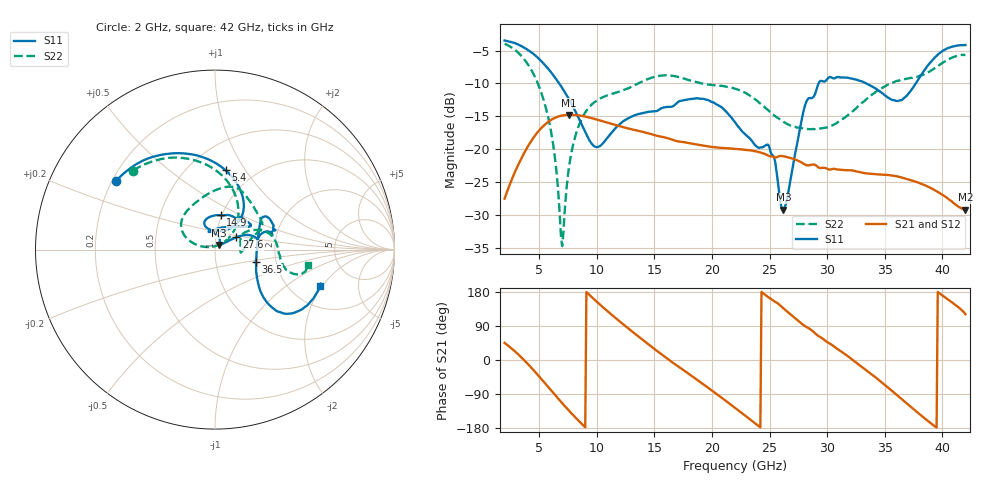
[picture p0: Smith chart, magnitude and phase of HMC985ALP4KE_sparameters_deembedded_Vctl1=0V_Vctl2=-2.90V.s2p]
!s2p File: Measurements: S11, S21, S12, S22
# GHz S dB R 50.0
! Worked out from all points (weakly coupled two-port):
!   401 points, 2 GHz to 42 GHz, reference 50 ohm
!   highest |S21| = -14.78 dB at 7.6 GHz (marker M1); lowest = -29.2 dB at 42 GHz (marker M2)
!   lowest |S11| = -29.2 dB at 26.2 GHz (marker M3), VSWR 1.07, Z = 52.3 + j2.72 ohm
!   |S11| at or under -10 dB: 6.736 GHz to 29.26 GHz (22.52 GHz wide, 125 % of centre); 33.39 GHz to 37.7 GHz (4.308 GHz wide, 12.1 % of centre)
!   |S22| runs from -34.8 to -4.0 dB; largest |S21 - S12| = 0.00076
!   S11 on the Smith chart (normalised r, x): 2 GHz: 0.22, +0.30; 5.4 GHz: 0.74, +0.82; 14.9 GHz: 0.99, +0.39; 27.6 GHz: 1.26, +0.18; 36.5 GHz: 1.57, -0.22; 42 GHz: 2.92, -1.90
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2  -3.47 145.0  -27.53 45.1  -27.52 45.1  -3.97 136.0
3.5  -4.37 118.8  -21.26 5.5  -21.27 5.4  -5.92 102.0
5.4  -7.01 82.5  -16.42 -57.7  -16.44 -57.7  -12.61 56.2
6.3  -8.92 66.5  -15.29 -89.6  -15.27 -89.6  -20.36 40.1
6.9  -10.44 57.8  -14.92 -110.6  -14.94 -110.6  -33.41 74.2
7.1  -10.97 55.5  -14.85 -117.4  -14.88 -117.5  -32.70 138.1
7.6  -12.43 51.3  -14.78 -134.1  -14.80 -134.1  -22.62 166.5
8.7  -16.29 53.1  -14.94 -168.7  -14.93 -168.7  -15.36 157.9
10.1  -19.66 88.9  -15.56 151.0  -15.54 151.1  -12.48 142.7
14.9  -14.25 80.4  -17.79 31.5  -17.76 31.6  -9.07 81.0
15.4  -14.01 74.2  -18.05 20.2  -18.06 20.2  -8.86 76.5
19.3  -12.37 33.7  -19.47 -65.1  -19.48 -65.1  -10.04 42.9
22  -15.90 52.1  -19.95 -126.2  -19.98 -126.3  -10.80 25.0
25  -19.80 99.4  -21.07 163.7  -21.04 163.7  -14.28 13.1
26.2  -29.22 48.7  -21.07 136.4  -21.12 136.4  -15.83 1.5
27.6  -17.23 30.0  -21.86 100.3  -21.86 100.2  -16.74 -6.1
28.7  -12.21 13.0  -22.32 77.2  -22.33 77.1  -16.94 -1.4
31  -9.05 23.3  -23.12 27.0  -23.11 27.0  -15.81 26.1
35.4  -12.27 11.9  -23.95 -75.7  -23.93 -75.7  -10.12 16.9
36.5  -12.51 -16.4  -24.32 -104.0  -24.36 -104.0  -9.42 9.7
39.5  -5.83 -43.4  -26.41 -178.3  -26.35 -178.5  -7.46 -16.1
42  -4.15 -18.8  -29.21 120.7  -29.20 120.5  -5.64 -9.1
